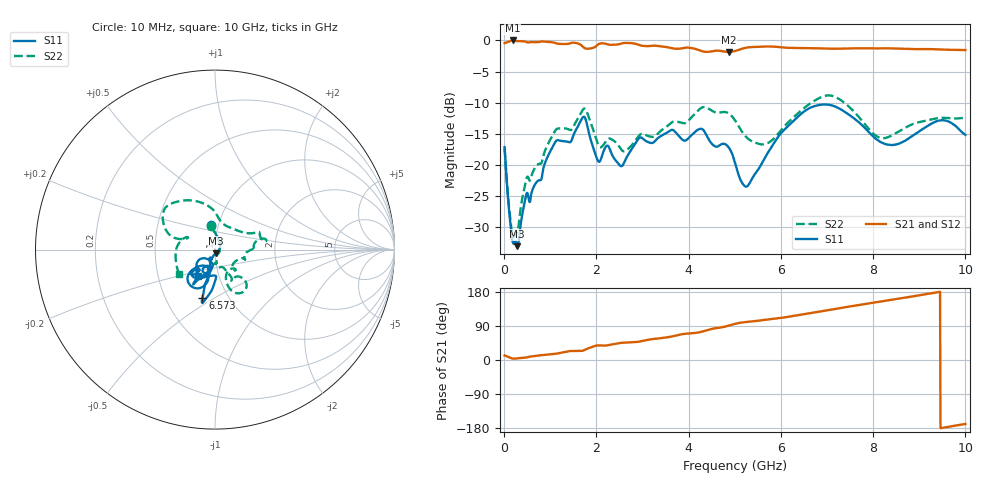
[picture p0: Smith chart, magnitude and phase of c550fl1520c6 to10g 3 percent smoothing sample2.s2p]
!Agilent Technologies,N5234A,MY52241123,A.10.00.00
!Agilent N5234A: A.10.00.00
!Date: Wednesday, April 24, 2019 09:07:22
!Correction: S11(Full 2 Port(1,2))
!S21(Full 2 Port(1,2))
!S12(Full 2 Port(1,2))
!S22(Full 2 Port(1,2))
!S2P File: Measurements: S11, S21, S12, S22:
# Hz S  dB  R 50
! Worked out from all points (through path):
!   1001 points, 10 MHz to 10 GHz, reference 50 ohm
!   highest |S21| = -0.01 dB at 189.8 MHz (marker M1); lowest = -1.9 dB at 4.865 GHz (marker M2)
!   lowest |S11| = -33.1 dB at 279.7 MHz (marker M3), VSWR 1.05, Z = 50.7 - j2.13 ohm
!   |S11| at or under -10 dB: start of sweep to end of sweep
!   |S22| runs from -31.7 to -8.8 dB; largest |S21 - S12| = 0.0021
!   S11 on the Smith chart (normalised r, x): 10 MHz: 0.93, +0.26; 6.573 GHz: 0.76, -0.44; 10 GHz: 0.79, -0.24
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1e7  -17.16 98.3  -0.44 12.1  -0.43 12.2  -17.41 99.4
1.8982e8  -32.50 -3.7  -0.01 3.7  -0.00 3.8  -31.54 5.6
2.7973e8  -33.08 -71.2  -0.11 4.3  -0.11 4.3  -30.84 -52.6
4.8952e8  -24.60 -115.6  -0.28 6.8  -0.28 6.8  -22.08 -86.2
1.09891e9  -16.46 -106.2  -0.38 16.0  -0.38 16.0  -14.62 -59.8
1.67833e9  -12.68 -112.2  -0.81 24.0  -0.81 24.0  -11.49 -48.6
2.04796e9  -19.49 -120.6  -0.60 38.5  -0.60 38.5  -16.91 -61.5
2.23777e9  -16.91 -115.0  -0.63 38.6  -0.62 38.6  -15.92 -44.0
2.54746e9  -20.21 -110.5  -0.49 45.5  -0.49 45.5  -17.63 -41.5
2.92708e9  -15.70 -117.8  -0.73 48.4  -0.73 48.4  -15.28 -16.9
3.34666e9  -15.63 -127.6  -0.91 56.8  -0.90 56.8  -14.87 -3.8
4.26574e9  -14.20 -128.9  -1.69 74.1  -1.68 74.1  -10.88 12.1
4.86514e9  -17.17 -138.2  -1.85 90.7  -1.85 90.7  -11.73 22.0
5.005e9  -19.70 -147.5  -1.70 95.4  -1.70 95.4  -12.84 23.6
5.27473e9  -23.44 -120.3  -1.14 100.6  -1.14 100.6  -15.72 40.7
5.73427e9  -17.86 -103.5  -0.98 106.9  -0.98 107.0  -16.43 72.4
6.57343e9  -11.08 -104.6  -1.26 122.4  -1.25 122.4  -10.47 114.3
6.67333e9  -10.71 -104.5  -1.27 124.4  -1.26 124.4  -9.95 120.2
7.24276e9  -10.86 -101.4  -1.33 136.2  -1.33 136.2  -9.34 148.6
8.34166e9  -16.78 -89.9  -1.27 157.6  -1.28 157.6  -15.50 155.7
9.45055e9  -12.86 -121.8  -1.46 179.9  -1.46 179.9  -12.45 -148.8
1e10  -15.19 -123.2  -1.55 -169.0  -1.55 -169.1  -12.43 -146.0
